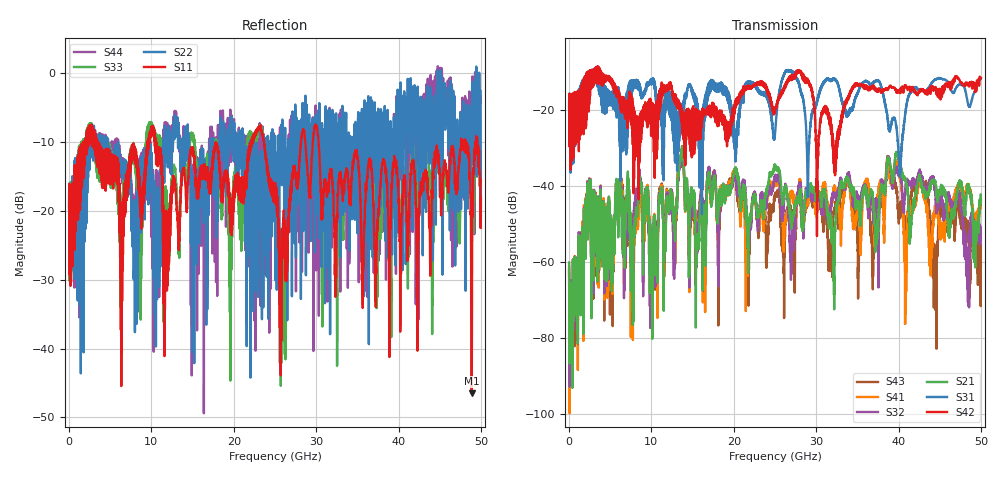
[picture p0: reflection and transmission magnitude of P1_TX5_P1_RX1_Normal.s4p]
!Keysight Technologies,N5225B,MY57041031,A.13.20.10
!Date: Friday, May 31, 2019 11:14:08
!Correction: S11(Full 4 Port(1,2,3,4))
!S12(Full 4 Port(1,2,3,4))
!S13(Full 4 Port(1,2,3,4))
!S14(Full 4 Port(1,2,3,4))
!S21(Full 4 Port(1,2,3,4))
!S22(Full 4 Port(1,2,3,4))
!S23(Full 4 Port(1,2,3,4))
!S24(Full 4 Port(1,2,3,4))
!S31(Full 4 Port(1,2,3,4))
!S32(Full 4 Port(1,2,3,4))
!S33(Full 4 Port(1,2,3,4))
!S34(Full 4 Port(1,2,3,4))
!S41(Full 4 Port(1,2,3,4))
!S42(Full 4 Port(1,2,3,4))
!S43(Full 4 Port(1,2,3,4))
!S44(Full 4 Port(1,2,3,4))
!S4P File: Measurements: <S11,S12,S13,S14>,
!<S21,S22,S23,S24>,
!<S31,S32,S33,S34>,
!<S41,S42,S43,S44>:
# Hz S  dB  R 50.0
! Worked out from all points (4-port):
!   5000 points, 10 MHz to 50 GHz, reference 50 ohm
!   strongest paths, dB at 10 MHz, 12.51 GHz, 25.01 GHz, 37.51 GHz, 50 GHz:
!     S42: -19.5, -14.8, -20.0, -14.9, -11.6
!     S31: -19.3, -23.2, -26.1, -12.3, -11.7
!     S21: -60.2, -42.5, -35.1, -51.1, -43.7
!     S32: -62.1, -42.2, -37.6, -55.6, -53.9
!     S41: -61.3, -42.2, -39.4, -42.7, -44.4
!     S43: -63.0, -42.5, -42.3, -47.8, -60.7
!   lowest |S11| = -46.5 dB at 48.89 GHz (marker M1), VSWR 1.01, Z = 49.5 - j0.0472 ohm
!   |S11| at or under -10 dB: 3.502 GHz to 9.556 GHz (6.054 GHz wide, 92.7 % of centre); 10.5 GHz to 22.11 GHz (11.6 GHz wide, 71.2 % of centre); 30.29 GHz to 47.6 GHz (17.31 GHz wide, 44.4 % of centre)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
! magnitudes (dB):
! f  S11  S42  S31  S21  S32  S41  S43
! 10 MHz  -19.8  -19.5  -19.3  -60.2  -62.1  -61.3  -63.0
! 2.35 GHz  -10.6  -18.9  -13.3  -42.7  -42.2  -42.5  -42.0
! 10 GHz  -7.9  -23.2  -13.0  -61.6  -59.4  -56.3  -55.3
! 13.67 GHz  -15.5  -22.8  -22.7  -30.5  -31.9  -30.5  -32.1
! 15.57 GHz  -18.0  -20.4  -22.6  -54.2  -57.0  -49.6  -50.4
! 48.89 GHz  -46.5  -12.9  -17.4  -44.7  -47.8  -43.3  -49.1
! 50 GHz  -18.2  -11.6  -11.7  -43.7  -53.9  -44.4  -60.7
